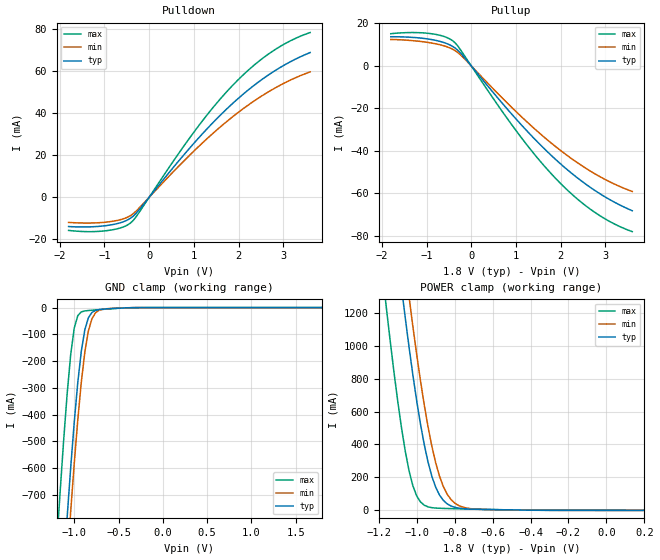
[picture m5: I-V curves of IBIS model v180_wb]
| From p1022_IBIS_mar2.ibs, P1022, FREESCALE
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|   Model v180_wb
[Model]   v180_wb
Model_type   I/O
Polarity   Non-Inverting
Enable   Active-High
Vinl =   0.63V
Vinh =   1.17V
Vmeas =  0.9000V
Cref =   0.0F
Rref =   50.0000
Vref =   0.9000V
C_comp   3.0088pF   2.9071pF   3.0187pF
[Temperature Range]   85.0000   0.1250k   -40.0000
[Voltage Range]   1.8000V   1.6200V   1.9800V
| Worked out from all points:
|   slope of the pulldown table from 0 to 0.27 V, typ, clamps not added: 37.7 ohm
|   slope of the pullup table from 0 to 0.27 V, typ, clamps not added: 38.8 ohm
|   GND clamp passes 1 mA (typ) near -0.40 V on its own axis
|   POWER clamp passes 1 mA (typ) near -0.37 V on its own axis
[Pulldown]
|Voltage   I(typ)   I(min)   I(max)
-1.8V     -13.88mA   -11.92mA   -15.72mA
-960mV    -13.44mA   -11.78mA   -15.87mA
-660mV    -12.18mA   -10.72mA   -14.65mA
-420mV    -9.968mA   -8.714mA   -12.27mA
-240mV    -6.338mA   -5.45mA    -7.688mA
1.02V     26.17mA    22.4mA     31.55mA
1.44V     35.82mA    30.68mA    43mA
1.8V      43.35mA    37.18mA    51.74mA
2.28V     52.16mA    44.86mA    61.66mA
2.7V      58.68mA    50.6mA     68.63mA
3.12V     64.06mA    55.38mA    74.03mA
3.6V      68.88mA    59.7mA     78.4mA
[Pullup]
|Voltage   I(typ)   I(min)   I(max)
-1.8V     13.74mA    12.45mA    15.18mA
-960mV    12.66mA    11.03mA    15.35mA
-660mV    11.32mA    9.756mA    14.2mA
-420mV    9.224mA    7.887mA    11.92mA
-240mV    6.083mA    5.212mA    7.553mA
1.02V     -25.47mA   -21.92mA   -31.03mA
1.44V     -34.96mA   -30.11mA   -42.38mA
1.86V     -43.59mA   -37.59mA   -52.44mA
2.28V     -51.22mA   -44.27mA   -61.05mA
2.7V      -57.8mA    -50.06mA   -68.1mA
3.12V     -63.29mA   -54.88mA   -73.61mA
3.6V      -68.25mA   -59.18mA   -78.11mA
[GND_clamp]
|Voltage   I(typ)   I(min)   I(max)
-1.8V     -4.804A    -4.965A    -4.352A
-1.2V     -1.391A    -1.566A    -898mA
-1.16V    -1.182A    -1.356A    -692.5mA
-1.08V    -783mA     -952.3mA   -322.2mA
-1.04V    -598.3mA   -762.1mA   -175.8mA
-1V       -428.7mA   -583.2mA   -76.41mA
-920mV    -162.7mA   -278.3mA   -16.12mA
-880mV    -82.2mA    -165.4mA   -12.47mA
-840mV    -37.92mA   -87mA      -10.97mA
-800mV    -18.2mA    -41.64mA   -9.843mA
-720mV    -7.422mA   -10.26mA   -7.766mA
1.8V      9.036uA    41.65uA    11.05uA
[POWER_clamp]
|Voltage   I(typ)   I(min)   I(max)
-1.8V     9.621A     9.869A     8.815A
-1.16V    2.159A     2.491A     1.232A
-1.08V    1.354A     1.674A     501.9mA
-1.06V    1.168A     1.482A     358.5mA
-1.04V    989.9mA    1.296A     239.6mA
-1V       666mA      947mA      88.04mA
-960mV    399.2mA    640.1mA    31.27mA
-920mV    207mA      389.6mA    16.4mA
-880mV    93.61mA    209mA      12.71mA
-840mV    40.16mA    99.64mA    11.19mA
-780mV    13.9mA     30.06mA    9.524mA
200mV     0A         0A         0A
[Ramp]
| variable   typ   min   max
dV/dt_r  0.6027/0.3566n   0.5062/0.4989n   0.7208/0.2171n
dV/dt_f  0.6105/0.3135n   0.5122/0.4426n   0.7259/0.2039n
R_load = 50.0000
|End [Model] v180_wb
